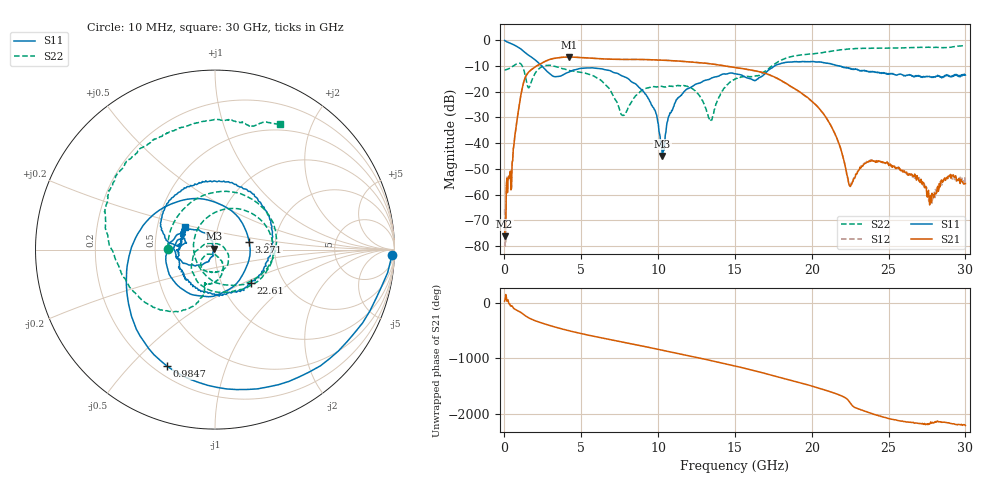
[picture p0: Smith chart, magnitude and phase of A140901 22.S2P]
!  2-Port S-parameters saved by WinCal
! VAR MeasName=S-Parameters (CALIBRATED_DATA) read from VNA (N5244A)
! VAR MeasDate=11/3/2014 9:28:38 AM
! VAR NAME=A140901 22
! VAR FILENAME=A140901 22.S2P
! VAR DATE=11/3/2014 9:28:38 AM
! VAR PHYS_PORTS=1,2
# Hz S RI R 50
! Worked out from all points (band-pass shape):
!   801 points, 10 MHz to 30 GHz, reference 50 ohm
!   highest |S21| = -6.55 dB at 4.209 GHz (marker M1); lowest = -76.2 dB at 10 MHz (marker M2)
!   |S21| within 3 dB of the highest: 2.23 GHz to 13.85 GHz (11.62 GHz wide, 145 % of centre)
!   lowest |S11| = -45.0 dB at 10.28 GHz (marker M3), VSWR 1.01, Z = 49.6 + j0.429 ohm
!   |S11| at or under -10 dB: 2.427 GHz to 17.58 GHz (15.16 GHz wide, 151 % of centre); 21.76513 GHz to 21.8274 GHz (62.27 MHz wide, 0.286 % of centre); 21.83 GHz to end of sweep
!   |S22| runs from -31.5 to -2.1 dB; largest |S21 - S12| = 0.0041
!   S11 on the Smith chart (normalised r, x): 10 MHz: 22, -53; 984.7 MHz: 0.25, -0.64; 3.271 GHz: 1.46, +0.14; 22.61 GHz: 1.37, -0.55; 30 GHz: 0.69, +0.18
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1e7  0.9862 -0.0314  0.000137 7.2e-05  -0.00017 -0.000486  -0.2645 0.00611
4.973375e8  0.4126 -0.734  0.0019 -0.0037  0.00182 -0.00373  -0.0874 0.2913
9.84675e8  -0.2679 -0.6487  -0.0572 -0.0191  -0.0573 -0.019  0.3248 0.1481
1.584475e9  -0.4923 -0.1205  0.018 0.2408  0.0181 0.2408  -0.1182 -0.00766
2.221762e9  -0.2653 0.2445  0.3232 0.0751  0.3227 0.075  0.1669 0.218
3.271412e9  0.1904 0.0445  0.1026 -0.4338  0.103 -0.4334  0.2821 -0.1289
4.2086e9  0.0517 -0.2351  -0.3844 -0.2709  -0.3845 -0.2711  0.123 -0.226
5.033325e9  -0.1539 -0.2392  -0.4373 0.1421  -0.4372 0.1426  0.00447 -0.2359
6.3079e9  -0.2736 -0.046  0.0145 0.4353  0.0143 0.4349  -0.1319 -0.0967
7.769912e9  -0.1648 0.107  0.4178 0.0611  0.4169 0.0615  0.0121 0.0331
1.001916e10  -0.0105 0.0203  -0.1928 -0.3653  -0.1924 -0.3644  0.00896 -0.1248
1.028158e10  -0.00358 0.00432  -0.278 -0.2997  -0.277 -0.2993  0.00111 -0.1256
1.121876e10  -0.032 -0.0627  -0.3919 0.0471  -0.3919 0.0469  -0.0374 -0.1241
1.343052e10  -0.1623 -0.0781  0.2593 0.2287  0.2604 0.2292  -0.00361 -0.0276
1.5005e10  -0.2207 0.0309  0.1636 -0.2447  0.1599 -0.2452  0.00923 -0.1758
1.665445e10  -0.1911 0.0183  -0.236 -0.0537  -0.2346 -0.0514  -0.055 -0.2065
2.002832e10  0.0741 0.3785  0.0357 -0.0535  0.0362 -0.0529  -0.5291 -0.1087
2.137788e10  0.3148 0.1164  -0.0183 -0.0022  -0.0182 -0.00236  -0.6094 0.1126
2.261496e10  0.1988 -0.1871  0.00127 -0.000993  0.00137 -0.00107  -0.5712 0.3559
2.501416e10  -0.1833 -0.1158  0.000458 0.00364  0.00064 0.00379  -0.2664 0.6509
2.775075e10  -0.1816 0.0605  0.000891 0.000356  0.000702 0.000109  0.1065 0.7156
3e10  -0.167 0.1267  0.00122 -0.00109  0.00128 -0.000986  0.3618 0.6992
